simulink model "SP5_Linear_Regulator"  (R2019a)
settings: Solver=VariableStepAuto  StartTime=0  StopTime=0.5  FixedStep=1e-5  RelTol=1e-5
libraries: fl_lib x6, nesl_utility x5, ee_lib x2

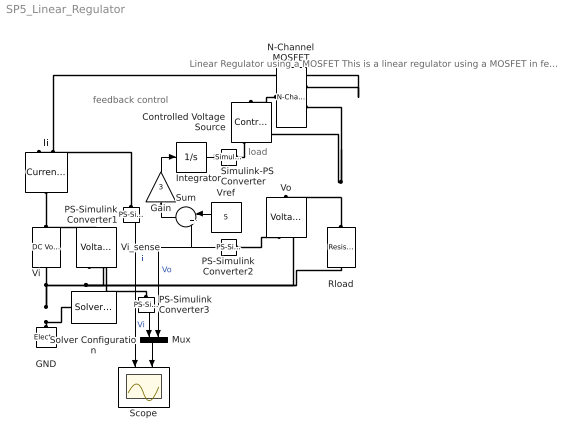
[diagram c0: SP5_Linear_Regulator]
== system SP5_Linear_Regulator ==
  note: Linear Regulator using a MOSFET This is a linear regulator using a MOSFET in feedback control with a resistive load. 1. Assume the input is a 9-V battery. Set the amplitude of Vi to 9 V (double click Vi). 2. Simulate the circuit (click the Run button above). 3. Open the Scope below (double click). Press the "Scale X & Y Axis Limits" to fit data to the screen. 4. Observe the current and voltage waveforms. 5. Notice that the feedback control drives the system to its final steady-state operating point. C1. Capture the two voltage and current waveforms. Q1. What is the steady-state input power? Q2. What is the steady-state output power? Q3. What is the efficiency of the linear regulator? ------------------------------------------------------- Let's say that the load now requires a higher voltage. 6. Change the reference voltage (Vref) to 8 to change the output voltage to 8 V. 7. Simulate the circuit again (click the Run button above). C3. Capture the new two voltage and current waveforms. Q4. What is the new steady-state input power? Q5. What is the new steady-state output power? Q6. What is the new efficiency of the linear regulator? Q7. What input and output conditions lead to high efficiency in the linear regulator? Explain briefly. _________________________________ Play: Try changing the gain value of the feedback control. Observe how the shape of the output voltage waveforms changes. Observe how changing the value affects how quickly the voltage converges to the reference value.
  note: load
  note: feedback control
  Controlled Voltage Source : fl_lib/Electrical/Electrical Sources/Controlled Voltage Source
  GND : fl_lib/Electrical/Electrical Elements/Electrical Reference
  Gain : Gain  Gain=3
  Ii : fl_lib/Electrical/Electrical Sensors/Current Sensor
  Integrator : Integrator
  Mux : Mux  Inputs=2
  N-Channel MOSFET : ee_lib/Semiconductors & Converters/N-Channel MOSFET  parameterization=1  prmDatasheet=1  prmEquCoeff=1  Beta=5.0 A/V^2  Rds=0.025 Ohm  Id=6.0 A  Vgs=10 V  Vth=1.7 V  lam=0 1/V  Tmeas=25 degC  RS=0.0001 Ohm  RD=0.01 Ohm  C_param=1  C_GS=270 pF  C_GD=80 pF  C_DS=0 pF  C_iss=350 pF  C_rss=80 pF  C_oss=0 pF  C_GS_vec=[270, 300, 290, 280, 295, 255] pF  C_GD_vec=[450, 400, 300, 190, 95, 55] pF  C_DS_vec=[450, 410, 390, 230, 175, 115] pF  C_iss_vec=[720, 700, 590, 470, 390, 310] pF  C_rss_vec=[450, 400, 300, 190, 95, 55] pF  C_oss_vec=[900, 810, 690, 420, 270, 170] pF  C_Vds_vec=[.1, .3, 1, 3, 10, 30] V  V_GS_for_cap_data=0 V  charge_linearity_param=1  C_OX=200 pF  V_C_OX=-0.5 V  IsDiode=0 A  Vbi=0.6 V  n=1  Cj0Diode=0 pF  TT=50e-9 s  dVth_dT=-6 mV/K  Rds_T2=0.037 Ohm  Tmeas2=125 degC  BEXDatasheet=-1.5  BEXEquCoeff=-1.5  etaisDatasheet=3  etaisEquCoeff=3  TdeviceDatasheet=25 degC  TdeviceEquCoeff=25 degC  Rth=[1, 10] K/W  thermal_mass_parameterization=1  thermal_mass=[1, 1] J/K  thermal_time_constant=[1, 10] s  thermal_mass_initial_temperatures=[25, 25] degC  betaref=18 A/V^2  Vfbref=-1.1 V  gamma=3.5 V^0.50000  phib2ref=1 V  thesatref=0.4 1/V  alpha=0  Vp=5e-2 V  thesrref=0 1/V  m=8  Tref=25 degC  Cox=1500 pF  Cgso=100 pF  Cgdo=14 pF  Rsref=2e-3 Ohm  Rdref=0.17 Ohm  Rgref=8.4 Ohm  Isref=5.2e-13 A  Cj0=480 pF  Tprm=1  etabet=1.3  Stvfb=5e-4 V/K  Stphib=-8.5e-4 V/K  etasat=1.04  etasr=0.65  etar=0.95  etais=3  Tsim=25 degC  T0=[25, 25] degC
  PS-Simulink Converter1 : nesl_utility/PS-Simulink Converter  PhysicalDomain=network_engine_domain  SubClassName=ps_output  LeftPortType=input  RightPortType=output  PseudoPeriodic=off  Frequencies=[]  Unit=1  AffineConversion=off
  PS-Simulink Converter2 : nesl_utility/PS-Simulink Converter  PhysicalDomain=network_engine_domain  SubClassName=ps_output  LeftPortType=input  RightPortType=output  PseudoPeriodic=off  Frequencies=[]  Unit=1  AffineConversion=off
  PS-Simulink Converter3 : nesl_utility/PS-Simulink Converter  PhysicalDomain=network_engine_domain  SubClassName=ps_output  LeftPortType=input  RightPortType=output  PseudoPeriodic=off  Frequencies=[]  Unit=1  AffineConversion=off
  Rload : ee_lib/Passive/Resistor  R=10 Ohm  R_tol=5  enable_R_tol=0  tol_distribution=1  nSigma=4  enable_operating_limits=0  operating_limit_action=2  max_working_voltage=100 V  power_rating=1 W  enable_faults=0  fault_action=1  R_faulted=inf Ohm  enable_temporal_fault=0  t_fault=1 s  enable_behavioral_fault=0  max_permissible_current=1 A  t_fail_on_current=1 s  noise_mode=0  sample_time=1e-3 s  repeatability=1  auto_seed=4267928862  user_seed=0  Tdevice=25 degC  alpha=3.93e-3 1/K  Tmeas=25 degC  thermal_mass=100 J/K  power_derating_T1=70 degC  power_derating_T2=155 degC  operating_temperature_range_vec=[-50, 150] degC  temperature_specify=off  temperature_priority=High  temperature=298.15 K  temperature_nominal_specify=off  temperature_nominal_unit=K  temperature_nominal_value=1
  Scope : Scope  NumInputPorts=2
  Simulink-PS Converter : nesl_utility/Simulink-PS Converter  PhysicalDomain=network_engine_domain  SubClassName=ps_input  LeftPortType=input  RightPortType=output  PseudoPeriodic=off  Frequencies=[]  NoiseDistribution=none  NoiseParameters=[]  Unit=1  AffineConversion=off  FilteringAndDerivatives=provide  SimscapeFilterOrder=1  InputFilterTimeConstant=0.001  UdotUserProvided=0
  Solver Configuration : nesl_utility/Solver Configuration  PhysicalDomain=network_engine_domain  SubClassName=solver  LeftPortType=input  RightPortType=generic  Tones=[]  Harmonics=[]  SimulateNoise=off  Profile=off  UseLocalSampling=off  EnableSwitchedLinearOptims=on  FrequencyDomain=off  UseCCode=off  RelTol=0.001  AbsTol=1e-06  MinStep=1e-09  ToWorkspace=off  RevertToSquareIcSolve=off  NumHomotopyIterations=100  PhasorMode=off  PhasorModeNumHarmonics=1  DoDC=off  ResidualTolerance=1e-09  UseLocalSolver=off  LocalSolverChoice=NE_BACKWARD_EULER_ADVANCER  LocalSolverSampleTime=0.001  DoFixedCost=off  MaxNonlinIter=3  MaxModeIter=2  LinearAlgebra=auto  EquationFormulation=NE_TIME_EF  DelaysMemoryBudget=1024  AutomaticFiltering=on  FilteringTimeConstant=0.001  PartitionStorageMethod=AS_NEEDED  PartitionMemoryBudget=1024  PartitionMethod=ROBUST
  Sum : Sum  Inputs=|+-
  Vi : fl_lib/Electrical/Electrical Sources/DC Voltage Source  v0=1 V
  Vi_sense : fl_lib/Electrical/Electrical Sensors/Voltage Sensor
  Vo : fl_lib/Electrical/Electrical Sensors/Voltage Sensor
  Vref : Constant  Value=5
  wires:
  PS-Simulink Converter2/1 -> Mux/2, Sum/2  "Vo"
  PS-Simulink Converter3/1 -> Mux/1  "Vi"
  Vref/1 -> Sum/1
  Integrator/1 -> Simulink-PS Converter/1
  Sum/1 -> Gain/1
  Mux/1 -> Scope/2
  PS-Simulink Converter1/1 -> Scope/1  "Ii"
  Gain/1 -> Integrator/1
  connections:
  GND/LConn1 -- Vi_sense/RConn2 -- Rload/RConn1 -- Vo/RConn2 -- Vi/RConn1 -- Solver Configuration/RConn1
  PS-Simulink Converter2/LConn1 -- Vo/RConn1
  Vi/LConn1 -- Vi_sense/LConn1 -- Ii/LConn1
  Ii/RConn2 -- N-Channel MOSFET/RConn1
  Vo/LConn1 -- Controlled Voltage Source/RConn2 -- N-Channel MOSFET/RConn2 -- Rload/LConn1
  N-Channel MOSFET/LConn1 -- Controlled Voltage Source/LConn1
  Controlled Voltage Source/RConn1 -- Simulink-PS Converter/RConn1
  PS-Simulink Converter3/LConn1 -- Vi_sense/RConn1
  PS-Simulink Converter1/LConn1 -- Ii/RConn1
